PROGRAM MAIN
VAR
	power1: MC_Power;
	axis1: AXIS_REF;
	power1_output:ST_McOutputs;
	
	move_abs: MC_MoveAbsolute;
	init_pos: LREAL;
	move_init_output:ST_McOutputs;
	
	SetPointGenEnable: MC_ExtSetPointGenEnable;
	SetPointGenDisable: MC_ExtSetPointGenDisable;
	SetPointGenEnable_output,SetPointGenDisable_output:ST_McOutputs;	
	enable,disable:BOOL;
	
	reset_output:ST_McOutputs;
	axis_Reset: MC_Reset;
	
	gen_state:state;
	
	position: LREAL;
	velocity: LREAL;
	direction: DINT;	
	acceleration: LREAL;
	t:lreal;
	

	
	
END_VAR

axis1();(*更新轴状态*)

power();
setpositionGen();
reset();
move_init();

CASE gen_state OF
	init:
		power1.Enable:=FALSE;
		SetPointGenEnable.Execute:=FALSE;
		SetPointGenDisable.Execute:=FALSE;
		axis_Reset.Execute:=FALSE;
		gen_state:=gen_power;
		init_pos:= SIN(0) + 2*COS(0) + 3*COS(0) + 4*COS(0);
		
	gen_power:
		power1.Enable:=TRUE;
		IF power1_output.Done THEN
			gen_state:=gen_move;
		END_IF
		IF axis1.Status.Error THEN
			gen_state := gen_error;
		END_IF
		
	gen_move:
		move_abs.Execute:=TRUE;
		IF move_abs.Done  THEN
			move_abs.Execute:=FALSE;
			gen_state:=gen_enable;
		END_IF
	
	gen_enable:
		setpointgenenable.Execute:=TRUE;
		IF SetPointGenEnable.Enabled THEN
			t:=t+0.01;
			MC_ExtSetPointGenFeed(
				Position:= SIN(2*t) + 2*COS(4*t) + 3*COS(2*t) + 4*COS(4*t), 		
				Velocity:= 2*COS(2*t)-8*SIN(4*t)-6*SIN(2*t)-16*SIN(4*t), 
				Acceleration:=-4*SIN(2*t)-32*COS(4*t)-12*COS(2*t)-64*COS(4*t) , 
				Direction:= 1,
				Axis:= axis1);		
		END_IF
		IF axis1.Status.Error THEN
			gen_state := gen_error;
		END_IF
	
	gen_error:
		SetPointGenEnable.Execute:=FALSE;
		SetPointGenDisable.Execute := SetPointGenEnable.Enabled;	
		IF NOT axis1.Status.Coupled THEN
			IF axis1.Status.Error THEN
				gen_state := gen_reset;	
			ELSE
				gen_state := init;
			END_IF
		END_IF
	
	gen_reset:
		axis_Reset.Execute := TRUE;
		SetPointGenDisable.Execute:=FALSE;
			
			IF axis_Reset.Done  THEN
				gen_state := init;
			ELSIF axis_Reset.Error  THEN
				gen_state := init; 
			END_IF
		
END_CASE

ACTION move_init:
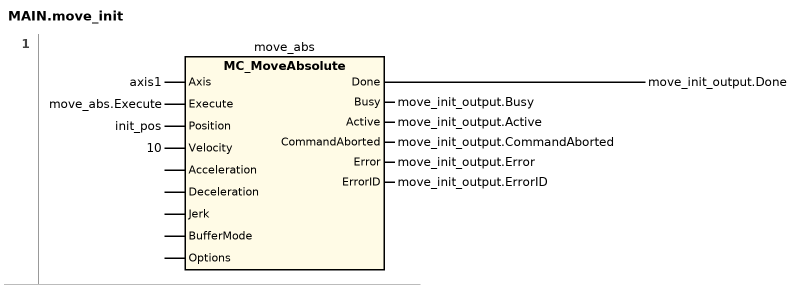
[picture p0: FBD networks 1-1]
// NETWORK 1
move_abs(
    Axis := axis1,
    Execute := move_abs.Execute,
    Position := init_pos,
    Velocity := 10,
    Busy => move_init_output.Busy,
    Active => move_init_output.Active,
    CommandAborted => move_init_output.CommandAborted,
    Error => move_init_output.Error,
    ErrorID => move_init_output.ErrorID); // MC_MoveAbsolute
move_init_output.Done := move_abs.Done;
END_ACTION

ACTION power:
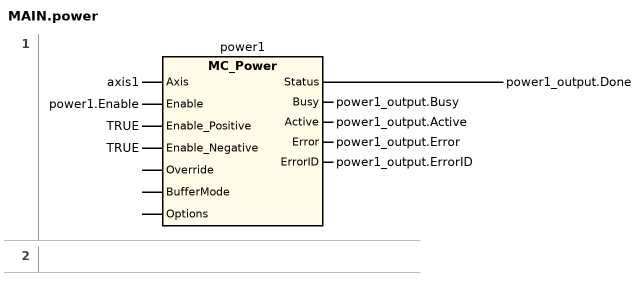
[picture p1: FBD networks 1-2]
// NETWORK 1
power1(
    Axis := axis1,
    Enable := power1.Enable,
    Enable_Positive := TRUE,
    Enable_Negative := TRUE,
    Busy => power1_output.Busy,
    Active => power1_output.Active,
    Error => power1_output.Error,
    ErrorID => power1_output.ErrorID); // MC_Power
power1_output.Done := power1.Status;

// NETWORK 2
END_ACTION

ACTION reset:
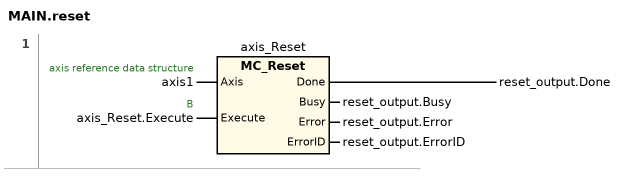
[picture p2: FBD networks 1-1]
// NETWORK 1
//   axis1: axis reference data structure
//   axis_Reset.Execute: B
axis_Reset(
    Axis := axis1,
    Execute := axis_Reset.Execute,
    Busy => reset_output.Busy,
    Error => reset_output.Error,
    ErrorID => reset_output.ErrorID); // MC_Reset
reset_output.Done := axis_Reset.Done;
END_ACTION

ACTION setpositionGen:
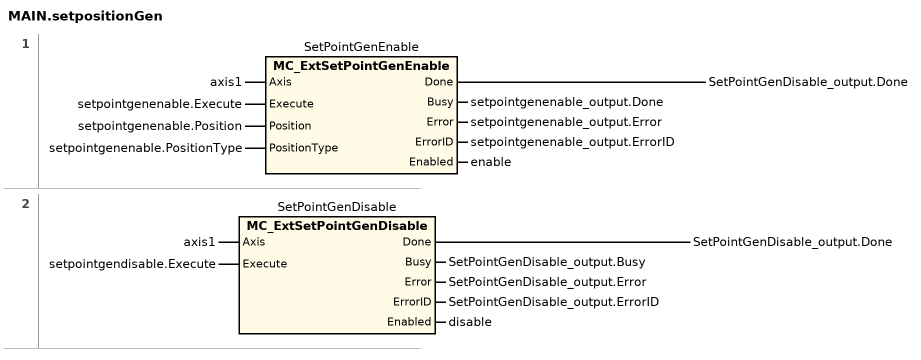
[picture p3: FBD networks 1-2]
// NETWORK 1
SetPointGenEnable(
    Axis := axis1,
    Execute := setpointgenenable.Execute,
    Position := setpointgenenable.Position,
    PositionType := setpointgenenable.PositionType,
    Busy => setpointgenenable_output.Done,
    Error => setpointgenenable_output.Error,
    ErrorID => setpointgenenable_output.ErrorID,
    Enabled => enable); // MC_ExtSetPointGenEnable
SetPointGenDisable_output.Done := SetPointGenEnable.Done;

// NETWORK 2
SetPointGenDisable(
    Axis := axis1,
    Execute := setpointgendisable.Execute,
    Busy => SetPointGenDisable_output.Busy,
    Error => SetPointGenDisable_output.Error,
    ErrorID => SetPointGenDisable_output.ErrorID,
    Enabled => disable); // MC_ExtSetPointGenDisable
SetPointGenDisable_output.Done := SetPointGenDisable.Done;
END_ACTION

END_PROGRAM
